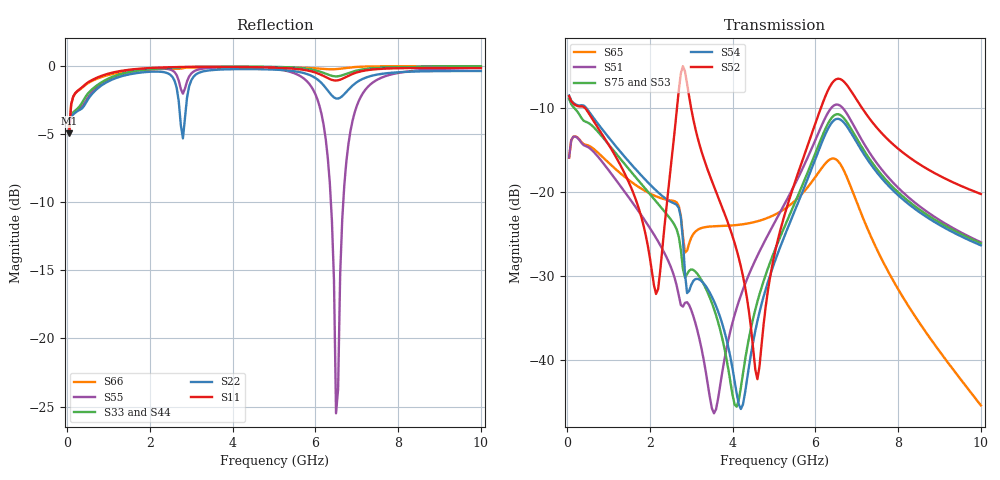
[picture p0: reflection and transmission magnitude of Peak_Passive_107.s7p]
! Created Tue Jun  9 06:58:47 2020
# ghz S ma R 50
! 7 Port Network Data from SP1.SP block
! freq  magS11  angS11  magS12  angS12  magS13  angS13  magS14  angS14
!  magS15  angS15  magS16  angS16  magS17  angS17
!  magS21  angS21
!  magS22  angS22  magS23  angS23  magS24  angS24  magS25  angS25
!  magS26  angS26  magS27  angS27
!  magS31  angS31  magS32  angS32
!  magS33  angS33  magS34  angS34  magS35  angS35  magS36  angS36
!  magS37  angS37
!  magS41  angS41  magS42  angS42  magS43  angS43
!  magS44  angS44  magS45  angS45  magS46  angS46  magS47  angS47
!  magS51  angS51  magS52  angS52  magS53  angS53  magS54  angS54
!  magS55  angS55  magS56  angS56  magS57  angS57
!  magS61  angS61
!  magS62  angS62  magS63  angS63  magS64  angS64  magS65  angS65
!  magS66  angS66  magS67  angS67
!  magS71  angS71  magS72  angS72
!  magS73  angS73  magS74  angS74  magS75  angS75  magS76  angS76
!  magS77  angS77
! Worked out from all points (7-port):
!   200 points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, 50 MHz to 10 GHz, reference 50 ohm
!   strongest paths, dB at 50 MHz, 2.55 GHz, 5.05 GHz, 7.55 GHz, 10 GHz:
!     S52: -8.6, -15.1, -26.6, -12.7, -20.3
!     S54: -8.6, -21.3, -27.9, -18.1, -26.4
!     S75: -8.9, -23.6, -26.6, -17.7, -26.1
!     S53: -8.9, -23.6, -26.6, -17.7, -26.1
!     S51: -15.9, -29.5, -23.3, -17.0, -26.0
!     S65: -15.9, -21.0, -22.6, -27.5, -45.4
!   lowest |S11| = -4.9 dB at 50 MHz (marker M1), VSWR 3.62, Z = 16.1 - j19.6 ohm
!   |S11| at or under -10 dB: nowhere
